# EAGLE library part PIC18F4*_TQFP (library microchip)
USB Microcontrollers with nanoWatt Technology High-Performance, Enhanced Flash, 28/40/44-Pin, Source: http://ww1.microchip.com/downloads/en/devicedoc/39632c.pdf
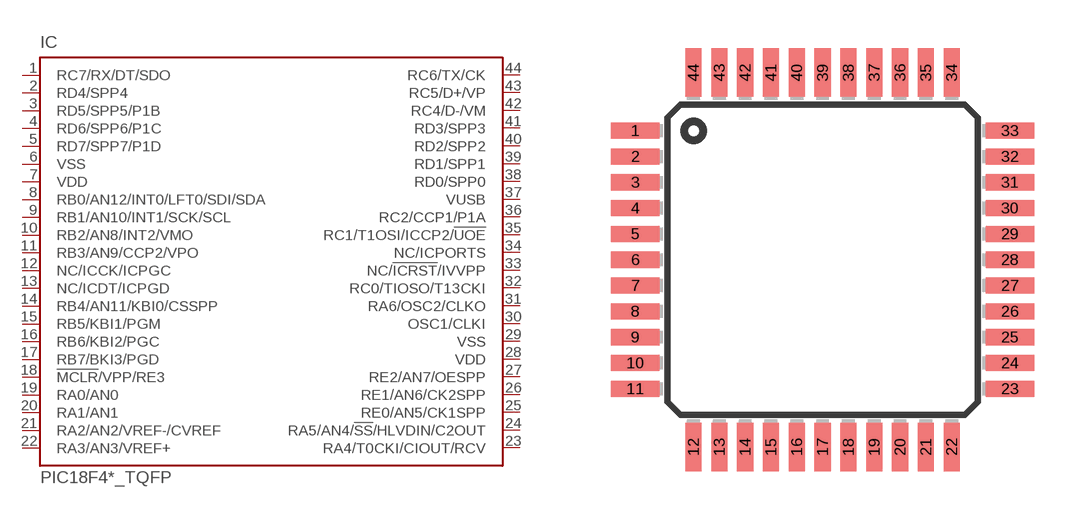
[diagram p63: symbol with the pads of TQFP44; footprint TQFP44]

Designator prefix IC

## PIC18F4455_TQFP (MF: MICROCHIP; MPN: PIC18F4455-I/PT; OC_FARNELL: 9321322; OC_NEWARK: 08J9628), PIC18F4550_TQFP (MF: MICROCHIP; MPN: PIC18F4550-I/PT; OC_FARNELL: 9321365; OC_NEWARK: 08J9633)  [TQFP44]
1  RC7/RX/DT/SDO
2  RD4/SPP4
3  RD5/SPP5/P1B
4  RD6/SPP6/P1C
5  RD7/SPP7/P1D
6  VSS  pwr
7  VDD  pwr
8  RB0/AN12/INT0/LFT0/SDI/SDA
9  RB1/AN10/INT1/SCK/SCL
10  RB2/AN8/INT2/VMO
11  RB3/AN9/CCP2/VPO
12  NC/ICCK/ICPGC
13  NC/ICDT/ICPGD
14  RB4/AN11/KBI0/CSSPP
15  RB5/KBI1/PGM
16  RB6/KBI2/PGC
17  RB7/BKI3/PGD
18  !MCLR!/VPP/RE3  in
19  RA0/AN0
20  RA1/AN1
21  RA2/AN2/VREF-/CVREF
22  RA3/AN3/VREF+
23  RA4/T0CKI/CIOUT/RCV
24  RA5/AN4/!SS!/HLVDIN/C2OUT
25  RE0/AN5/CK1SPP
26  RE1/AN6/CK2SPP
27  RE2/AN7/OESPP
28  VDD  pwr
29  VSS  pwr
30  OSC1/CLKI  in
31  RA6/OSC2/CLKO  out
32  RC0/TIOSO/T13CKI
33  NC/!ICRST!/IVVPP  in
34  NC/ICPORTS  in
35  RC1/T1OSI/ICCP2/!UOE
36  RC2/CCP1/P1A
37  VUSB
38  RD0/SPP0
39  RD1/SPP1
40  RD2/SPP2
41  RD3/SPP3
42  RC4/D-/VM
43  RC5/D+/VP
44  RC6/TX/CK

## Footprint TQFP44 (pad centres in mm)
Thin Quad Flat Pack package type TQ
smd 1.5 x 0.5: 1 -5.8,4; 2 -5.8,3.2; 3 -5.8,2.4; 4 -5.8,1.6; 5 -5.8,0.8; 6 -5.8,0; 7 -5.8,-0.8; 8 -5.8,-1.6; 9 -5.8,-2.4; 10 -5.8,-3.2; 11 -5.8,-4; 23 5.8,-4; 24 5.8,-3.2; 25 5.8,-2.4; 26 5.8,-1.6; 27 5.8,-0.8; 28 5.8,0; 29 5.8,0.8; 30 5.8,1.6; 31 5.8,2.4; 32 5.8,3.2; 33 5.8,4
smd 0.5 x 1.5: 12 -4,-5.8; 13 -3.2,-5.8; 14 -2.4,-5.8; 15 -1.6,-5.8; 16 -0.8,-5.8; 17 0,-5.8; 18 0.8,-5.8; 19 1.6,-5.8; 20 2.4,-5.8; 21 3.2,-5.8; 22 4,-5.8; 34 4,5.8; 35 3.2,5.8; 36 2.4,5.8; 37 1.6,5.8; 38 0.8,5.8; 39 0,5.8; 40 -0.8,5.8; 41 -1.6,5.8; 42 -2.4,5.8; 43 -3.2,5.8; 44 -4,5.8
